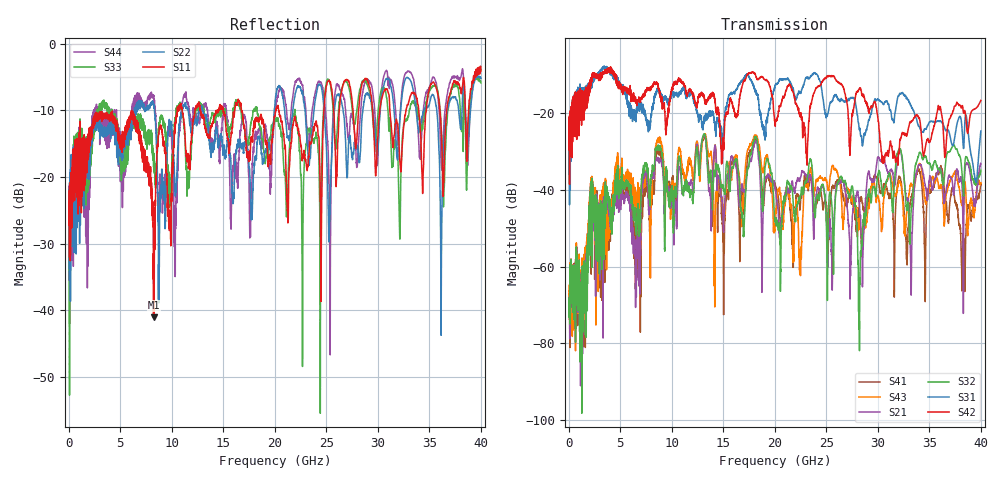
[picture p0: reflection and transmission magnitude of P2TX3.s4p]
!Agilent Technologies,N5245A,MY49151084,A.09.20.08
!Agilent N5245A: A.09.20.08
!Date: Thursday, March 01, 2012 11:52:55
!Correction: S11(Full 4 Port(1,2,3,4))
!S12(Full 4 Port(1,2,3,4))
!S13(Full 4 Port(1,2,3,4))
!S14(Full 4 Port(1,2,3,4))
!S21(Full 4 Port(1,2,3,4))
!S22(Full 4 Port(1,2,3,4))
!S23(Full 4 Port(1,2,3,4))
!S24(Full 4 Port(1,2,3,4))
!S31(Full 4 Port(1,2,3,4))
!S32(Full 4 Port(1,2,3,4))
!S33(Full 4 Port(1,2,3,4))
!S34(Full 4 Port(1,2,3,4))
!S41(Full 4 Port(1,2,3,4))
!S42(Full 4 Port(1,2,3,4))
!S43(Full 4 Port(1,2,3,4))
!S44(Full 4 Port(1,2,3,4))
!S4P File: Measurements: <S11,S12,S13,S14>,
!<S21,S22,S23,S24>,
!<S31,S32,S33,S34>,
!<S41,S42,S43,S44>:
# Hz S  dB  R 50
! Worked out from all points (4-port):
!   3996 points, 50 MHz to 40 GHz, reference 50 ohm
!   strongest paths, dB at 50 MHz, 10.04 GHz, 20.03 GHz, 30.02 GHz, 40 GHz:
!     S42: -23.6, -13.5, -22.7, -21.8, -16.7
!     S31: -25.5, -15.1, -12.9, -16.5, -24.7
!     S32: -69.6, -38.9, -47.6, -35.9, -34.9
!     S21: -69.5, -41.1, -39.5, -31.5, -33.2
!     S43: -64.9, -38.8, -49.0, -41.9, -38.1
!     S41: -66.3, -37.8, -38.5, -37.1, -38.5
!   lowest |S11| = -41.1 dB at 8.24 GHz (marker M1), VSWR 1.02, Z = 49.7 + j0.838 ohm
!   |S11| at or under -10 dB: start of sweep to 10.55 GHz; 16.77 GHz to 20.1 GHz (3.332 GHz wide, 18.1 % of centre); 20.38 GHz to 24.77 GHz (4.394 GHz wide, 19.5 % of centre)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
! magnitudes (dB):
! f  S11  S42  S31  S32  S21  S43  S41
! 50 MHz  -23.8  -23.6  -25.5  -69.6  -69.5  -64.9  -66.3
! 8.24 GHz  -41.1  -12.6  -17.6  -35.2  -36.7  -35.4  -38.6
! 26.45 GHz  -7.4  -12.4  -16.2  -36.6  -37.5  -41.5  -38.7
! 28.23 GHz  -8.3  -13.5  -24.2  -70.2  -44.4  -48.1  -43.0
! 32.05 GHz  -14.7  -30.5  -15.4  -29.5  -30.3  -37.7  -36.4
! 33.21 GHz  -7.7  -22.3  -18.0  -46.7  -61.0  -38.4  -42.7
! 40 GHz  -4.1  -16.7  -24.7  -34.9  -33.2  -38.1  -38.5
